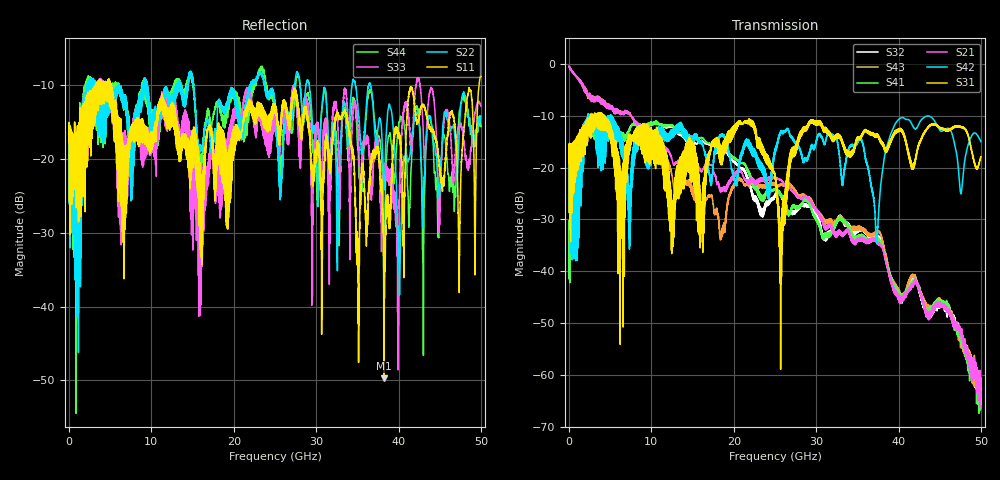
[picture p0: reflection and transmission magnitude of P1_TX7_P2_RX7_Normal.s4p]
!Keysight Technologies,N5225A,MY51441389,A.10.49.11
!Date: Monday, July 08, 2019 13:05:49
!Correction: S11(Full 4 Port(1,2,3,4))
!S12(Full 4 Port(1,2,3,4))
!S13(Full 4 Port(1,2,3,4))
!S14(Full 4 Port(1,2,3,4))
!S21(Full 4 Port(1,2,3,4))
!S22(Full 4 Port(1,2,3,4))
!S23(Full 4 Port(1,2,3,4))
!S24(Full 4 Port(1,2,3,4))
!S31(Full 4 Port(1,2,3,4))
!S32(Full 4 Port(1,2,3,4))
!S33(Full 4 Port(1,2,3,4))
!S34(Full 4 Port(1,2,3,4))
!S41(Full 4 Port(1,2,3,4))
!S42(Full 4 Port(1,2,3,4))
!S43(Full 4 Port(1,2,3,4))
!S44(Full 4 Port(1,2,3,4))
!S4P File: Measurements: <S11,S12,S13,S14>,
!<S21,S22,S23,S24>,
!<S31,S32,S33,S34>,
!<S41,S42,S43,S44>:
# Hz S  dB  R 50
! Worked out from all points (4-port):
!   5000 points, 10 MHz to 50 GHz, reference 50 ohm
!   strongest paths, dB at 10 MHz, 12.51 GHz, 25.01 GHz, 37.51 GHz, 50 GHz:
!     S31: -19.0, -28.8, -21.3, -14.1, -17.9
!     S42: -19.1, -13.3, -16.4, -31.0, -15.0
!     S21: -0.4, -18.4, -21.9, -34.6, -60.9
!     S41: -33.2, -11.8, -24.1, -33.9, -62.2
!     S43: -0.4, -21.6, -23.1, -32.4, -63.9
!     S32: -32.7, -12.0, -25.3, -33.4, -65.7
!   lowest |S11| = -49.7 dB at 38.23 GHz (marker M1), VSWR 1.01, Z = 50.3 - j0.0208 ohm
!   |S11| at or under -10 dB: start of sweep to 3.25 GHz; 3.252 GHz to 3.298 GHz (45.98 MHz wide, 1.4 % of centre); 5.103 GHz to 49.78 GHz (44.68 GHz wide, 163 % of centre)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
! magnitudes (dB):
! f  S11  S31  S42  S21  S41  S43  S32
! 10 MHz  -17.6  -19.0  -19.1  -0.4  -33.2  -0.4  -32.7
! 10.56 GHz  -15.8  -19.1  -15.7  -14.9  -11.0  -15.3  -11.1
! 22.1 GHz  -13.5  -10.8  -16.0  -22.7  -22.0  -23.1  -23.9
! 25.67 GHz  -16.3  -33.1  -13.4  -22.3  -25.1  -23.2  -24.9
! 36.56 GHz  -21.7  -13.3  -22.4  -34.4  -34.3  -33.3  -33.6
! 38.23 GHz  -49.7  -15.6  -18.6  -36.5  -36.4  -35.1  -35.7
! 50 GHz  -8.8  -17.9  -15.0  -60.9  -62.2  -63.9  -65.7
